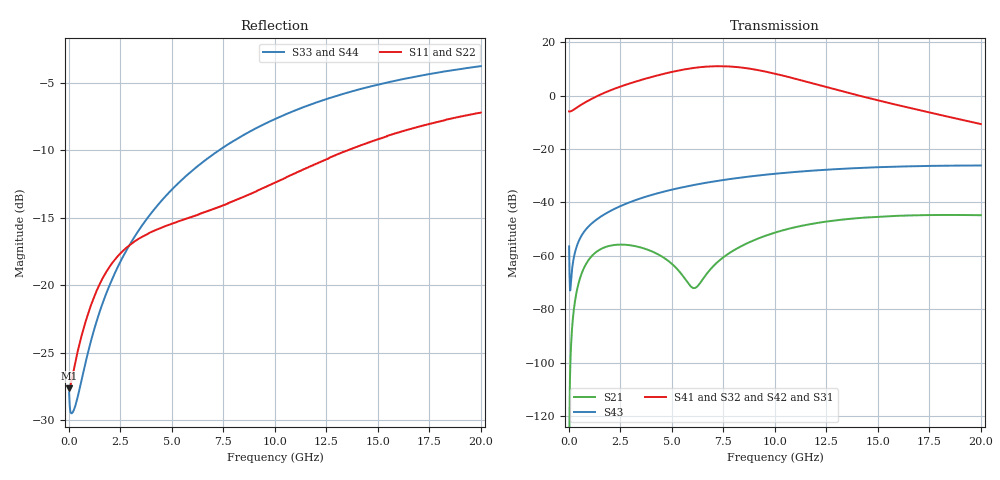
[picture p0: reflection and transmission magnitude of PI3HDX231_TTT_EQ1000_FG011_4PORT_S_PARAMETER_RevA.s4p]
! NPort=4 DATA=2000 NOISE=0 GROUPDELAY=0 COMPLEX_DATAFORMAT=POLAR
! NumOfBlock=1 NumOfParam=0
! .MODEL Smodel S TSTONEFILE=PI3HDX231_TTT_EQ1000_FG011_4PORT_S_PARAMETER_RevA.s4p TYPE=S
!  -- The above .MODEL line can be used for the S element in the netlist.
! The s parameter is extracted from the linear redriver, it is not bi-directional; only s(4,1)s(4,2) and s(3,1)s(3,2)
! should be the insertion loss
!Port definition:
!Port1 = input+
!Port2 = input-
!Port3 = output+
!Port4 = output-
# Hz S MA R  50
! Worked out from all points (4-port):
!   2000 points, 10 MHz to 20 GHz, reference 50 ohm
!   strongest paths, dB at 10 MHz, 5.01 GHz, 10.01 GHz, 15.01 GHz, 20 GHz:
!     S41: -5.9, 8.9, 8.2, -1.8, -10.7
!     S32: -5.9, 8.8, 8.1, -1.8, -10.6
!     S42: -5.9, 8.9, 8.1, -2.0, -10.8
!     S31: -5.9, 8.8, 8.0, -2.2, -11.0
!     S43: -56.5, -35.2, -29.3, -26.9, -26.2
!     S21: -134.8, -63.1, -51.3, -45.4, -44.8
!   lowest |S11| = -27.6 dB at 10 MHz (marker M1), VSWR 1.09, Z = 46 - j0.0776 ohm
!   |S11| at or under -10 dB: start of sweep to 13.55 GHz
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1e7  0.04152 -178.8  1.825e-07 -13.9  0 0.0  0 0.0
     1.825e-07 -14.0  0.04152 -178.8  0 0.0  0 0.0
     0.5042 -0.1  0.5042 179.9  0.04012 -3.2  0.0015 -70.3
     0.5042 179.9  0.5042 -0.1  0.0015 -70.3  0.04012 -3.2
4.52e9  0.1636 -140.6  0.0009614 -10.2  3.438e-10 -157.7  2.163e-10 -141.2
        0.0009635 -10.1  0.1636 -140.7  2.096e-10 -141.3  3.563e-10 -157.4
        2.482 -46.9  2.488 132.8  0.2065 -101.0  0.01559 64.1
        2.501 132.7  2.502 -46.2  0.01556 64.0  0.2066 -101.0
6.48e9  0.1853 -137.1  0.0003539 83.1  3.104e-09 139.8  1.642e-09 179.7
        0.0003543 81.9  0.1851 -137.3  1.591e-09 -179.4  3.231e-09 139.2
        3.393 -106.5  3.41 73.2  0.2851 -106.7  0.02269 53.0
        3.428 73.0  3.429 -105.7  0.02261 53.0  0.2852 -106.7
8.31e9  0.2095 -132.8  0.001481 98.0  1.249e-08 82.4  8.197e-09 134.6
        0.001471 97.6  0.2088 -133.0  7.998e-09 136.1  1.295e-08 80.9
        3.309 -169.1  3.348 10.7  0.3536 -111.5  0.02905 41.5
        3.361 10.2  3.349 -168.2  0.02894 41.6  0.3537 -111.5
1.073e10  0.2547 -128.8  0.003262 76.8  4.24e-08 17.2  3.435e-08 62.1
          0.003242 76.5  0.2532 -128.9  3.393e-08 63.9  4.331e-08 15.0
          2.13 118.6  2.185 -61.9  0.4356 -117.4  0.03645 25.7
          2.187 -62.5  2.162 119.7  0.03633 25.9  0.4357 -117.4
1.372e10  0.3197 -128.5  0.004972 45.9  1.172e-07 -49.3  9.53e-08 -16.3
          0.004939 45.7  0.3177 -128.5  9.541e-08 -14.6  1.179e-07 -51.5
          1.041 54.1  1.087 -127.6  0.5208 -124.0  0.04339 6.3
          1.082 -128.3  1.062 55.4  0.04332 6.5  0.5206 -124.0
2e10  0.4355 -135.6  0.005782 -4.3  3.803e-07 -161.0  2.823e-07 -139.5
      0.005737 -4.4  0.4338 -135.4  2.86e-07 -138.6  3.765e-07 -162.7
      0.2803 -44.0  0.2959 130.5  0.6464 -135.0  0.04884 -32.3
      0.292 130.1  0.2895 -42.6  0.04894 -32.1  0.6461 -135.0
